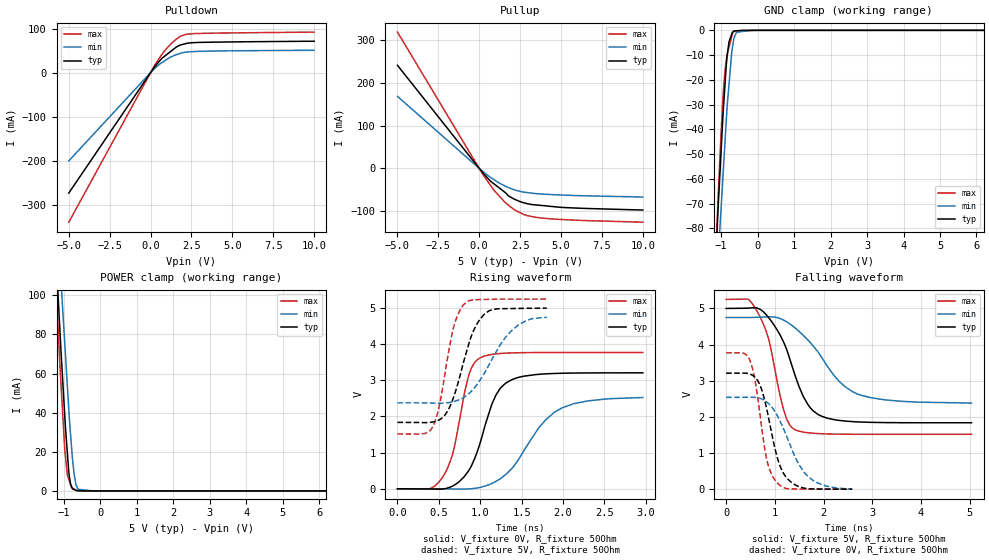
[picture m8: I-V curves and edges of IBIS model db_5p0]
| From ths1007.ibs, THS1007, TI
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|   db_5p0 Model
[Model]   db_5p0
Model_type   I/O
Polarity   Non-Inverting
Enable   Active-High
Vinl = 0.6
Vinh = 2.6
Vmeas = 2.5
Vref = 2.5
Cref = 30pF
Rref = 50
|   typ   min   max
|   (nom PVT)   (fast PVT)   (slow PVT)
C_comp   1.743e-12   1.734e-12   1.762e-12
|ON state : BUFFER OUTPUT TURNED HIGH
|C_comp   1.893e-12   1.883e-12   1.924e-12
|OFF state: BUFFER IN HIGH IMPEDANCE
|C_comp   1.593e-12   1.585e-12   1.601e-12
| Where nom  PVT is Nominal Process, 5V, 27C
| Fast PVT is Strong Process,  5.25V, -40C
| Slow PVT is Weak Process,   4.75V, 125C
[Voltage Range]   5   4.75   5.25
|Ambient Temperature   25   85   -40
|Junction Temperature
[Temperature Range]   27   125   -40
[Pullup Reference]   5   4.75   5.25
[Pulldown Reference]   0   0   0
[Power Clamp Reference]   5   4.75   5.25
[GND Clamp Reference]   0   0   0
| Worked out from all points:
|   slope of the pulldown table from 0 to 0.75 V, typ, clamps not added: 21.9 ohm
|   slope of the pullup table from 0 to 0.75 V, typ, clamps not added: 23.7 ohm
|   GND clamp passes 1 mA (typ) near -0.70 V on its own axis
|   POWER clamp passes 1 mA (typ) near -0.76 V on its own axis
|   falling waveform, V_fixture 5V, R_fixture 50Ohm: 20-80 % time 561ps typ, 858ps min, 383ps max; typ from 5 V to 1.84 V
|   rising waveform, V_fixture 0V, R_fixture 50Ohm: 20-80 % time 290ps typ, 490ps min, 211ps max; typ from 0 V to 3.21 V
|   rising waveform, V_fixture 5V, R_fixture 50Ohm: 20-80 % time 250ps typ, 386ps min, 181ps max; typ from 1.84 V to 5 V
|   falling waveform, V_fixture 0V, R_fixture 50Ohm: 20-80 % time 338ps typ, 529ps min, 254ps max; typ from 3.21 V to 0 V
[Pulldown]
|   Voltage   I(typ)   I(min)   I(max)
-5V       -273.8mA   -200.7mA   -340.2mA
278.2mV   14.45mA    10.34mA    18.49mA
700mV     32.81mA    23.07mA    41.84mA
924mV     39.34mA    28.46mA    52.67mA
1.292V    50.04mA    36.47mA    67.25mA
1.596V    58.91mA    41.32mA    76.89mA
1.848V    63.09mA    44.11mA    83.04mA
2.142V    65.97mA    46.51mA    87mA
2.635V    68.25mA    47.94mA    88.77mA
10V       71.52mA    50.93mA    92.28mA
[GND Clamp]
|   Voltage   I(typ)   I(min)   I(max)
-5V       -1.588A    -1.479A    -1.711A
-1.306V   -142.8mA   -157.4mA   -148.3mA
-1.088V   -73.23mA   -94.47mA   -69.17mA
-1.04V    -59.66mA   -81.53mA   -53.73mA
-1.008V   -50.58mA   -73.46mA   -43.33mA
-934.5mV  -30.74mA   -55.07mA   -23.72mA
-840mV    -10.96mA   -31.88mA   -9.869mA
-785mV    -4.686mA   -21.96mA   -6.794mA
-707.7mV  -1.417mA   -8.561mA   -2.476mA
-640mV    -254uA     -2.95mA    -291uA
-190mV    0A         -26.17nA   -86.38uA
10V       0A         0A         0A
[Pullup]
|   Voltage   I(typ)   I(min)   I(max)
-5V       240.8mA    168.3mA    318.4mA
288.8mV   -13.19mA   -9.295mA   -17.98mA
700mV     -30.18mA   -21.2mA    -40.11mA
924mV     -36.77mA   -26.8mA    -51.95mA
1.533V    -54.69mA   -40.35mA   -77.44mA
1.822V    -64.84mA   -45.16mA   -87.17mA
2.2V      -72.69mA   -50.69mA   -97.65mA
2.751V    -80.58mA   -55.49mA   -108.1mA
3.838V    -86.66mA   -59.79mA   -115.9mA
5.405V    -91.76mA   -62.72mA   -120mA
10V       -97.14mA   -66.87mA   -125.6mA
[POWER Clamp]
|   Voltage   I(typ)   I(min)   I(max)
-5V       1.67A      1.647A     1.704A
-1.306V   152.8mA    187.3mA    139.1mA
-1.103V   80.25mA    116.9mA    62.67mA
-1.08V    72.32mA    109.2mA    55.39mA
-1.026V   55.03mA    91.3mA     37.93mA
-971.2mV  37.5mA     74.56mA    20.54mA
-903mV    19.4mA     53.69mA    7.999mA
-855mV    8.251mA    39.01mA    5.399mA
-815mV    3.493mA    28.81mA    3.231mA
-722mV    738.4uA    9.286mA    1.048mA
-640mV    112.2uA    2.096mA    234.5uA
10V       0A         0A         0A
[Ramp]
R_load = 50
|   typ   min   max
dV/dt_r   1.9252/2.8943e-10   1.5242/4.90137e-10   2.26297/2.10078e-10
dV/dt_f   1.89789/5.57306e-10   1.42313/8.57476e-10   2.23902/3.82519e-10
[Falling Waveform]
V_fixture = 5V
V_fixture_min = 4.75V
V_fixture_max = 5.25V
R_fixture = 50Ohm
|   Time   V(typ)   V(min)   V(max)
0s        5V         4.75V      5.25V
440ps     5.008V     4.75V      5.26V
690ps     4.983V     4.759V     4.786V
890ps     4.717V     4.769V     4.062V
1.19ns    4.04V      4.672V     2.157V
1.41ns    3.171V     4.467V     1.649V
1.782ns   2.173V     3.971V     1.547V
2.262ns   1.914V     3.071V     1.523V
2.684ns   1.862V     2.641V     1.519V
5.038ns   1.837V     2.382V     1.519V
[Rising Waveform]
V_fixture = 0V
V_fixture_min = 0V
V_fixture_max = 0V
R_fixture = 50Ohm
|   Time   V(typ)   V(min)   V(max)
0s        1.848nV    2.664nV    1.618nV
380ps     -4.61mV    302.2uV    -4.877mV
548ps     -6.223mV   -2.56mV    330.7mV
672ps     82.22mV    -6.549mV   1.012V
858ps     494.7mV    -4.825mV   3.113V
1.002ns   1.293V     39.92mV    3.627V
1.186ns   2.574V     199.4mV    3.731V
1.388ns   3.025V     577.5mV    3.76V
1.988ns   3.197V     2.238V     3.771V
2.964ns   3.208V     2.525V     3.771V
[Rising Waveform]
V_fixture = 5V
V_fixture_min = 4.75V
V_fixture_max = 5.25V
R_fixture = 50Ohm
|   Time   V(typ)   V(min)   V(max)
0s        1.837V     2.378V     1.518V
430ps     1.849V     2.37V      1.735V
510ps     1.913V     2.367V     2.348V
628ps     2.25V      2.387V     3.912V
702ps     2.697V     2.427V     4.649V
798ps     3.502V     2.523V     5.091V
938ps     4.465V     2.816V     5.23V
1.11ns    4.928V     3.448V     5.243V
1.462ns   4.99V      4.537V     5.249V
1.804ns   4.999V     4.742V     5.25V
[Falling Waveform]
V_fixture = 0V
V_fixture_min = 0V
V_fixture_max = 0V
R_fixture = 50Ohm
|   Time   V(typ)   V(min)   V(max)
0s        3.209V     2.54V      3.772V
484ps     3.188V     2.544V     3.576V
608ps     3.074V     2.538V     2.903V
718ps     2.8V       2.503V     1.829V
840ps     2.177V     2.404V     788.3mV
1.06ns    829.3mV    2.013V     160.7mV
1.262ns   285.1mV    1.396V     13.87mV
1.634ns   20.43mV    416.6mV    1.873mV
2.042ns   2.899mV    91.01mV    495.6uV
2.588ns   201.6uV    1.309mV    177.9uV
